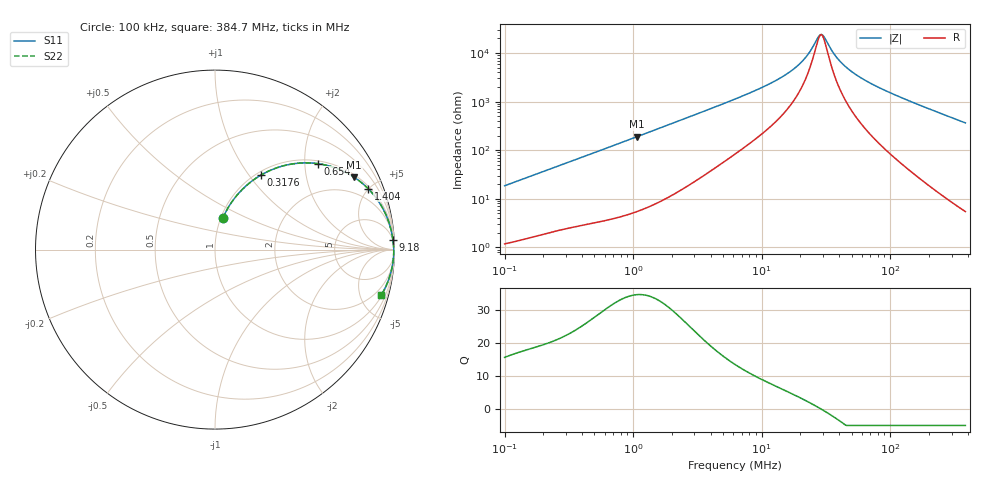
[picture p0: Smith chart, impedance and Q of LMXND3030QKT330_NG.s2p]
! LMXND3030QKT330_NG  S-PARAMETER MODEL  ( General Type )
! Model Generated by TAIYO YUDEN Corporation (http://www.ty-top.com)
! Version 1.0
! TAIYO YUDEN Control No. 200915NI43SB-FBB
! Copyright(c) 2020 TAIYO YUDEN CO.,LTD. All Rights Reserved.
! Product Description (link to TY-COMPAS)
! https://ds.yuden.co.jp/TYCOMPAS/or/detail?pn=LMXND3030QKT330MNG&u=M
! Products Name : Inductors
! Characteristics :
!  Inductance : 33 uH , SRF(min) : 18 MHz , DC Resistance(max) : 0.936 Ohm
!  Rated Current : Saturation :400 mA , Temp Rise : 440 mA
!  Case Size : 3.0 x 3.0 / 0.118 x 0.118 [mm/inch] , Thickness : 1.5 / 0.059 [mm/inch]
!  (Conditions: Temperature = 25 degC , DC Bias Current/Voltage = 0A / 0V)
! External Node Assignments :
!  1  o---GGG---o  2
! GND o---------o GND
! Frequency Range : 0.1MHz  -  384.651195MHz  [ 402 STEP ]
# MHz S RI R 50
! Freq[MHz].  S11 Real  S11 Imag  S21 Real  S21 Imag  S12 Real  S12 Imag  S22 Real  S22 Imag
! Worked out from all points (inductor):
!   401 points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, 100 kHz to 384.7 MHz, reference 50 ohm
!   read as one part in series: L = 29.2 uH near 104.2 kHz
!   highest Q = 34.8 at 1.073 MHz (marker M1), where L = 28.1 uH
!   self-resonance near 28.56 MHz
!   S11 on the Smith chart (normalised r, x): 100 kHz: 1.02, +0.37; 317.6 kHz: 1.05, +1.14; 654 kHz: 1.07, +2.32; 1.404 MHz: 1.15, +4.96; 9.18 MHz: 5, +35; 384.7 MHz: 1.11, -7.28
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0.1  0.0434 0.1744  0.9566 -0.1744  0.9566 -0.1744  0.0434 0.1744
0.185729  0.115 0.2941  0.885 -0.2941  0.885 -0.2941  0.115 0.2941
0.317621  0.2548 0.4145  0.7452 -0.4145  0.7452 -0.4145  0.2548 0.4145
0.398565  0.3425 0.4551  0.6575 -0.4551  0.6575 -0.4551  0.3425 0.4551
0.654038  0.5714 0.4791  0.4286 -0.4791  0.4286 -0.4791  0.5714 0.4791
1.073265  0.7761 0.4028  0.2239 -0.4028  0.2239 -0.4028  0.7761 0.4028
1.403529  0.853 0.3398  0.147 -0.3398  0.147 -0.3398  0.853 0.3398
1.588538  0.8801 0.31  0.1199 -0.31  0.1199 -0.31  0.8801 0.31
2.773253  0.9532 0.1922  0.0468 -0.1922  0.0468 -0.1922  0.9532 0.1922
6.331348  0.9863 0.0848  0.0137 -0.0848  0.0137 -0.0848  0.9863 0.0848
9.17961  0.991 0.056  0.00897 -0.056  0.00897 -0.056  0.991 0.056
13.30921  0.9936 0.0343  0.00635 -0.0343  0.00635 -0.0343  0.9936 0.0343
17.40472  0.9948 0.0215  0.00521 -0.0215  0.00521 -0.0215  0.9948 0.0215
21.39408  0.9954 0.0125  0.00462 -0.0125  0.00462 -0.0125  0.9954 0.0125
24.71908  0.9957 0.00652  0.00434 -0.00652  0.00434 -0.00652  0.9957 0.00652
27.97746  0.9958 0.00147  0.00417 -0.00147  0.00417 -0.00147  0.9958 0.00147
29.76434  0.9959 -0.00106  0.00411 0.00106  0.00411 0.00106  0.9959 -0.00106
37.34957  0.996 -0.0105  0.00403 0.0105  0.00403 0.0105  0.996 -0.0105
45.91053  0.9958 -0.0195  0.00418 0.0195  0.00418 0.0195  0.9958 -0.0195
62.56801  0.9951 -0.0349  0.0049 0.0349  0.0049 0.0349  0.9951 -0.0349
98.5215  0.9923 -0.0638  0.0077 0.0638  0.0077 0.0638  0.9923 -0.0638
384.6512  0.9266 -0.2535  0.0734 0.2535  0.0734 0.2535  0.9266 -0.2535
